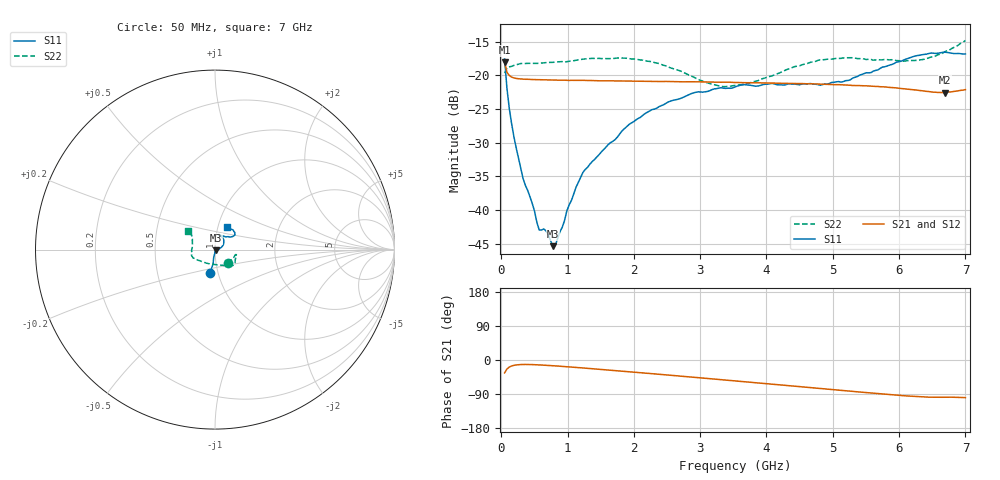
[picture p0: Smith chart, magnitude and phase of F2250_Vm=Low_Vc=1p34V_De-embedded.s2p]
! Integrated Device Technology
! Corporate Headquarters
! 6024 Silver Creek Valley Road
! San Jose, CA 95138  USA
! Phone:  1-408-284-8200
! Toll Free:  1-800-223-1366
! Webpage:  http://www.idt.com/
! Timing and RF Division
! 515 Groton Road, Suite 102
! Westford, MA 01886-6024
! Device:  F2250
! Description: Voltage Variable RF Attenuator
! Frequency:  50.0 -  6000.00 MHz
! Package:  3x3 mm Thin QFN Plastic Package: 16 pin
! Ports:  2 RF, 3 DC
!  Pin  1  = GND
!  Pin  2  = NC
!  Pin  3  = RF1  = Port 1
!  Pin  4  = NC
!  Pin  5  = GND
!  Pin  6  = GND
!  Pin  7  = GND
!  Pin  8  = GND
!  Pin  9  = NC
!  Pin 10  = RF2  = Port 2
!  Pin 11  = NC
!  Pin 12  = GND
!  Pin 13  = GND
!  Pin 14  = VCNTRL
!  Pin 15  = VDD
!  Pin 16  = VMODE
! Vcntrl:  1.340 Volts
! Vmode:  +0.000 Volts
! Vdd:  +3.30  Volts
! Current:  1.195 mA
! Data:  The device was measured on a the F2250 evaluation board which has
!  individual transmission lines to the RF pins.  Data was collected
!  using a calibrated network analyzer.  The evaluation board was
!  de-embedded using a TRL calibration technique.
!  The reference plane is the edge of the package pin.
! Misc:  SN 10
!  Action Tracker AT0258
! Date Measured:  2014-11-26
! Date:  2015-10-15  MJV
! Note:
!  Integrated Device Technology supplies this data as a sample of measured
!  data at the package pin for this product.  Your particular data for this
!  product may vary.
!  Data was taken at 25 degrees C.
!  Integrated Device Technology reserves the right to change this data at anytime.
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# GHz S dB R 50
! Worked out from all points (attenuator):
!   201 points, 50 MHz to 7 GHz, reference 50 ohm
!   highest |S21| = -18.06 dB at 50 MHz (marker M1); lowest = -22.6 dB at 6.687 GHz (marker M2)
!   lowest |S11| = -45.4 dB at 779.8 MHz (marker M3), VSWR 1.01, Z = 50.4 - j0.32 ohm
!   |S11| at or under -10 dB: start of sweep to end of sweep
!   |S22| runs from -21.7 to -14.8 dB; largest |S21 - S12| = 0.00033
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0.05  -17.58 -102.2  -18.06 -33.9  -18.06 -33.9  -19.70 -47.6
0.08475  -21.90 -97.5  -19.55 -23.9  -19.53 -23.9  -18.91 -24.1
0.15425  -27.11 -99.6  -20.26 -15.8  -20.27 -15.8  -18.68 -14.7
0.328  -35.33 -93.4  -20.58 -11.8  -20.58 -11.8  -18.25 -13.1
0.467  -39.04 -91.5  -20.64 -12.1  -20.64 -12.1  -18.26 -14.7
0.57125  -42.97 -73.9  -20.67 -12.9  -20.68 -12.9  -18.23 -17.3
0.6755  -43.13 -60.3  -20.71 -13.9  -20.69 -14.0  -18.13 -19.7
0.77975  -45.38 -36.1  -20.72 -15.1  -20.71 -15.1  -18.09 -22.3
0.8145  -45.26 -29.2  -20.72 -15.5  -20.72 -15.5  -18.05 -23.2
0.9535  -41.60 -23.7  -20.73 -17.3  -20.74 -17.3  -18.06 -26.6
0.98825  -40.15 -18.6  -20.75 -17.7  -20.75 -17.7  -17.98 -27.1
1.2315  -34.43 1.5  -20.76 -21.0  -20.76 -21.0  -17.60 -31.9
1.9265  -27.32 23.6  -20.87 -31.0  -20.87 -31.0  -17.53 -41.6
2.37825  -24.68 34.0  -20.94 -37.6  -20.93 -37.6  -18.26 -48.8
3.1775  -22.14 56.2  -21.01 -49.8  -21.02 -49.8  -21.33 -80.7
3.525  -21.75 66.0  -21.08 -55.1  -21.08 -55.1  -21.51 -105.1
4.7065  -21.33 69.1  -21.29 -73.5  -21.29 -73.5  -18.03 -156.9
5.22775  -20.78 52.5  -21.47 -81.7  -21.47 -81.7  -17.41 -165.8
5.85325  -18.51 37.1  -21.81 -91.3  -21.80 -91.4  -17.72 -178.3
6.33975  -16.97 38.7  -22.30 -97.3  -22.30 -97.3  -17.70 163.9
6.68725  -16.58 47.1  -22.57 -98.2  -22.56 -98.3  -16.52 149.4
7  -16.84 62.7  -22.13 -99.3  -22.13 -99.3  -14.84 145.6
